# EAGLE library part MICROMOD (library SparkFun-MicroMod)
MicroMod Connector Description: A card edge connector and mating PCB connector to allow various MicroMod Processor Boards to be coupled with various carrier boards of different capabilities. Based on the M.2 standard.
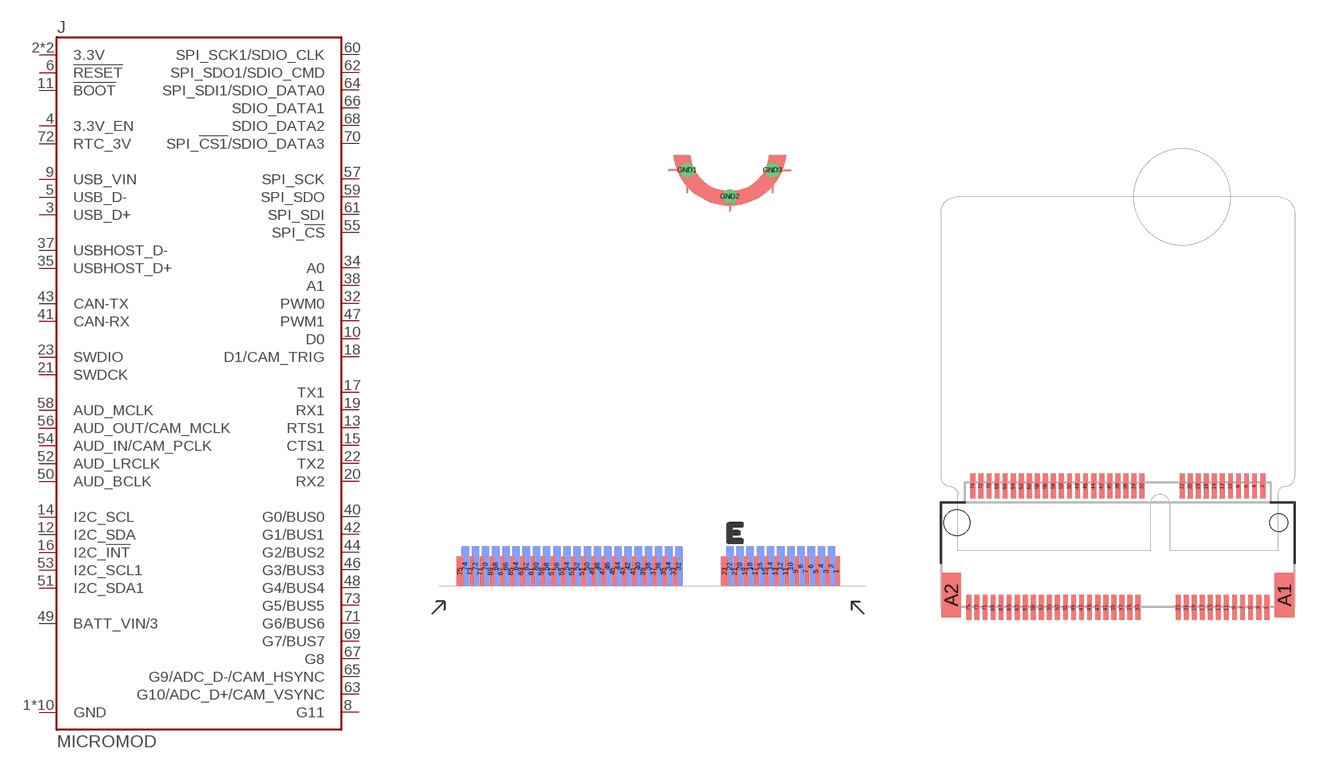
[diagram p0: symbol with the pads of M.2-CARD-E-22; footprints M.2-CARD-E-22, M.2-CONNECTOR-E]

Designator prefix J

## MICROMOD-2222  [M.2-CARD-E-22]
1  GND
2  3.3V
3  USB_D+
4  3.3V_EN
5  USB_D-
6  !RESET!
7  GND
8  G11
9  USB_VIN
10  D0
11  !BOOT!
12  I2C_SDA
13  RTS1
14  I2C_SCL
15  CTS1
16  I2C_!INT!
17  TX1
18  D1/CAM_TRIG
19  RX1
20  RX2
21  SWDCK
22  TX2
23  SWDIO
32  PWM0
33  GND
34  A0
35  USBHOST_D+
36  GND
37  USBHOST_D-
38  A1
39  GND
40  G0/BUS0
41  CAN-RX
42  G1/BUS1
43  CAN-TX
44  G2/BUS2
45  GND
46  G3/BUS3
47  PWM1
48  G4/BUS4
49  BATT_VIN/3
50  AUD_BCLK
51  I2C_SDA1
52  AUD_LRCLK
53  I2C_SCL1
54  AUD_IN/CAM_PCLK
55  SPI_!CS!
56  AUD_OUT/CAM_MCLK
57  SPI_SCK
58  AUD_MCLK
59  SPI_SDO
60  SPI_SCK1/SDIO_CLK
61  SPI_SDI
62  SPI_SDO1/SDIO_CMD
63  G10/ADC_D+/CAM_VSYNC
64  SPI_SDI1/SDIO_DATA0
65  G9/ADC_D-/CAM_HSYNC
66  SDIO_DATA1
67  G8
68  SDIO_DATA2
69  G7/BUS7
70  SPI_!CS1!/SDIO_DATA3
71  G6/BUS6
72  RTC_3V
73  G5/BUS5
74  3.3V
75  GND
GND1  GND
GND2  GND
GND3  GND

## MICROMOD-2222-C (PROD_ID: CONN-14877)  [M.2-CONNECTOR-E]
1  GND
2  3.3V
3  USB_D+
4  3.3V_EN
5  USB_D-
6  !RESET!
7  GND
8  G11
9  USB_VIN
10  D0
11  !BOOT!
12  I2C_SDA
13  RTS1
14  I2C_SCL
15  CTS1
16  I2C_!INT!
17  TX1
18  D1/CAM_TRIG
19  RX1
20  RX2
21  SWDCK
22  TX2
23  SWDIO
32  PWM0
33  GND
34  A0
35  USBHOST_D+
36  GND
37  USBHOST_D-
38  A1
39  GND
40  G0/BUS0
41  CAN-RX
42  G1/BUS1
43  CAN-TX
44  G2/BUS2
45  GND
46  G3/BUS3
47  PWM1
48  G4/BUS4
49  BATT_VIN/3
50  AUD_BCLK
51  I2C_SDA1
52  AUD_LRCLK
53  I2C_SCL1
54  AUD_IN/CAM_PCLK
55  SPI_!CS!
56  AUD_OUT/CAM_MCLK
57  SPI_SCK
58  AUD_MCLK
59  SPI_SDO
60  SPI_SCK1/SDIO_CLK
61  SPI_SDI
62  SPI_SDO1/SDIO_CMD
63  G10/ADC_D+/CAM_VSYNC
64  SPI_SDI1/SDIO_DATA0
65  G9/ADC_D-/CAM_HSYNC
66  SDIO_DATA1
67  G8
68  SDIO_DATA2
69  G7/BUS7
70  SPI_!CS1!/SDIO_DATA3
71  G6/BUS6
72  RTC_3V
73  G5/BUS5
74  3.3V
75  GND

## Footprint M.2-CARD-E-22 (pad centres in mm)
smd 0.35 x 1.45: 1 9.25,1.275; 3 8.75,1.275; 5 8.25,1.275; 7 7.75,1.275; 9 7.25,1.275; 11 6.75,1.275; 13 6.25,1.275; 15 5.75,1.275; 17 5.25,1.275; 19 4.75,1.275; 21 4.25,1.275; 23 3.75,1.275; 33 1.25,1.275; 35 0.75,1.275; 37 0.25,1.275; 39 -0.25,1.275; 41 -0.75,1.275; 43 -1.25,1.275; 45 -1.75,1.275; 47 -2.25,1.275; 49 -2.75,1.275; 51 -3.25,1.275; 53 -3.75,1.275; 55 -4.25,1.275; 57 -4.75,1.275; 59 -5.25,1.275; 61 -5.75,1.275; 63 -6.25,1.275; 65 -6.75,1.275; 67 -7.25,1.275; 69 -7.75,1.275; 71 -8.25,1.275; 73 -8.75,1.275; 75 -9.25,1.275
smd 0.35 x 1.95 bottom: 2 9,1.525; 4 8.5,1.525; 6 8,1.525; 8 7.5,1.525; 10 7,1.525; 12 6.5,1.525; 14 6,1.525; 16 5.5,1.525; 18 5,1.525; 20 4.5,1.525; 22 4,1.525; 32 1.5,1.525; 34 1,1.525; 36 0.5,1.525; 38 0,1.525; 40 -0.5,1.525; 42 -1,1.525; 44 -1.5,1.525; 46 -2,1.525; 48 -2.5,1.525; 50 -3,1.525; 52 -3.5,1.525; 54 -4,1.525; 56 -4.5,1.525; 58 -5,1.525; 60 -5.5,1.525; 62 -6,1.525; 64 -6.5,1.525; 66 -7,1.525; 68 -7.5,1.525; 70 -8,1.525; 72 -8.5,1.525; 74 -9,1.525
drill 0.2: GND1 1.9,21; GND2 4,19.7; GND3 6.1,21

## Footprint M.2-CONNECTOR-E (pad centres in mm)
smd 0.3 x 1.55: 1 9.25,-5.275; 2 9,2.275; 3 8.75,-5.275; 4 8.5,2.275; 5 8.25,-5.275; 6 8,2.275; 7 7.75,-5.275; 8 7.5,2.275; 9 7.25,-5.275; 10 7,2.275; 11 6.75,-5.275; 12 6.5,2.275; 13 6.25,-5.275; 14 6,2.275; 15 5.75,-5.275; 16 5.5,2.275; 17 5.25,-5.275; 18 5,2.275; 19 4.75,-5.275; 20 4.5,2.275; 21 4.25,-5.275; 22 4,2.275; 23 3.75,-5.275; 32 1.5,2.275; 33 1.25,-5.275; 34 1,2.275; 35 0.75,-5.275; 36 0.5,2.275; 37 0.25,-5.275; 38 0,2.275; 39 -0.25,-5.275; 40 -0.5,2.275; 41 -0.75,-5.275; 42 -1,2.275; 43 -1.25,-5.275; 44 -1.5,2.275; 45 -1.75,-5.275; 46 -2,2.275; 47 -2.25,-5.275; 48 -2.5,2.275; 49 -2.75,-5.275; 50 -3,2.275; 51 -3.25,-5.275; 52 -3.5,2.275; 53 -3.75,-5.275; 54 -4,2.275; 55 -4.25,-5.275; 56 -4.5,2.275; 57 -4.75,-5.275; 58 -5,2.275; 59 -5.25,-5.275; 60 -5.5,2.275; 61 -5.75,-5.275; 62 -6,2.275; 63 -6.25,-5.275; 64 -6.5,2.275; 65 -6.75,-5.275; 66 -7,2.275; 67 -7.25,-5.275; 68 -7.5,2.275; 69 -7.75,-5.275; 70 -8,2.275; 71 -8.25,-5.275; 72 -8.5,2.275; 73 -8.75,-5.275; 74 -9,2.275; 75 -9.25,-5.275
smd 1.2 x 2.75: A1 10.35,-4.5; A2 -10.35,-4.5
hole 1.1 at 10,0
hole 1.6 at -10,0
